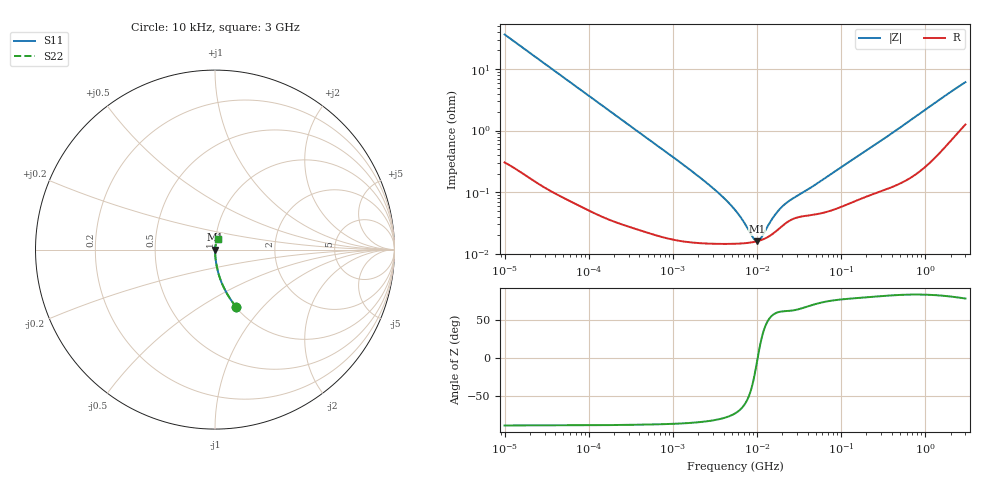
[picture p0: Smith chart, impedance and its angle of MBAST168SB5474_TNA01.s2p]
! MBAST168SB5474_TNA01  S-PARAMETER MODEL  ( Standard Model )
! Model Generated by TAIYO YUDEN Corporation (http://www.ty-top.com)
! Version 1.0
! TAIYO YUDEN Control No. 220601
! Copyright(c) 2012 TAIYO YUDEN CO.,LTD. All Rights Reserved.
! Product Description (link to TY-COMPAS)
! https://ds.yuden.co.jp/TYCOMPAS/or/detail?pn=MBAST168SB5474KTNA01&u=M
! Products Name : Multilayer Ceramic Capacitors
! Characteristics :
!  Capacitance : 0.47 [uF] , Rated Voltage : 25 [V] , TCC : X5R
!  Case Size : 1.6 x 0.8 / 0.063 x 0.031 [mm/inch] , Thickness : 0.8 / 0.031 [mm/inch]
!  (Conditions: Temperature = 25 [degC] , DC Bias Voltage = 0 [V])
! External Node Assignments :
!  1  o---| |---o  2
! GND o---------o GND
! Frequency Range : 10kHz  -  3GHz  [ 401 STEP ]
# MHZ S RI R 50
! Freq[MHz].  S11 Real  S11 Imag  S21 Real  S21 Imag  S12 Real  S12 Imag  S22 Real  S22 Imag
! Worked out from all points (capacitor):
!   401 points, 10 kHz to 3 GHz, reference 50 ohm
!   read as one part in series: C = 436 nF near 10.65 kHz
!   lowest |Z| = 15.9 mohm at 9.971 MHz (marker M1)
!   series resonance near 10.21 MHz, so ESL is about 560 pH
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0.01  0.1191 -0.3198  0.8809 0.3198  0.8809 0.3198  0.1191 -0.3198
0.015549  0.054 -0.2217  0.946 0.2217  0.946 0.2217  0.054 -0.2217
0.026575  0.0199 -0.1349  0.9801 0.1349  0.9801 0.1349  0.0199 -0.1349
0.045421  0.00734 -0.0802  0.9927 0.0802  0.9927 0.0802  0.00734 -0.0802
0.082683  0.00255 -0.0444  0.9974 0.0444  0.9974 0.0444  0.00255 -0.0444
0.199902  0.000674 -0.0185  0.9993 0.0185  0.9993 0.0185  0.000674 -0.0185
0.683653  0.000222 -0.00545  0.9998 0.00545  0.9998 0.00545  0.000222 -0.00545
2.737278  0.000147 -0.00128  0.9999 0.00128  0.9999 0.00128  0.000147 -0.00128
4.124064  0.000144 -0.000768  0.9999 0.000768  0.9999 0.000768  0.000144 -0.000768
5.477226  0.000145 -0.000494  0.9999 0.000494  0.9999 0.000494  0.000145 -0.000494
6.829836  0.000147 -0.000308  0.9999 0.000308  0.9999 0.000308  0.000147 -0.000308
9.070798  0.000154 -8.89e-05  0.9998 8.89e-05  0.9998 8.89e-05  0.000154 -8.89e-05
9.97066  0.000158 -1.76e-05  0.9998 1.76e-05  0.9998 1.76e-05  0.000158 -1.76e-05
10.61963  0.000162 3e-05  0.9998 -3e-05  0.9998 -3e-05  0.000162 3e-05
11.31085  0.000167 7.78e-05  0.9998 -7.78e-05  0.9998 -7.78e-05  0.000167 7.78e-05
15.50326  0.000211 0.000321  0.9998 -0.000321  0.9998 -0.000321  0.000211 0.000321
19.95104  0.000281 0.00051  0.9997 -0.00051  0.9997 -0.00051  0.000281 0.00051
24.87798  0.000348 0.000654  0.9997 -0.000654  0.9997 -0.000654  0.000348 0.000654
45.28751  0.000427 0.00114  0.9996 -0.00114  0.9996 -0.00114  0.000427 0.00114
374.4521  0.00123 0.00837  0.9988 -0.00837  0.9988 -0.00837  0.00123 0.00837
1755.269  0.00686 0.0366  0.9931 -0.0366  0.9931 -0.0366  0.00686 0.0366
3000  0.0158 0.0582  0.9842 -0.0582  0.9842 -0.0582  0.0158 0.0582
